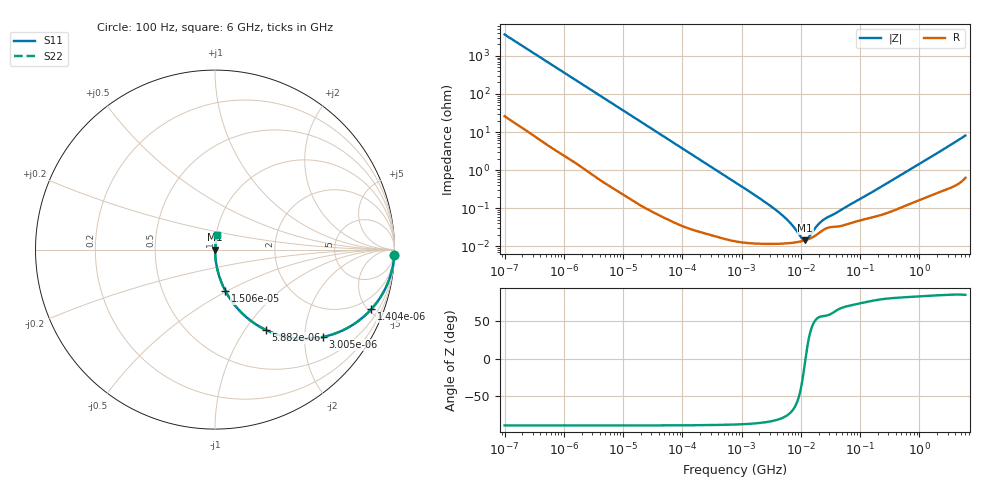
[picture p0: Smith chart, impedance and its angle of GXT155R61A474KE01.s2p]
!Murata Part Number: GXT155R61A474KE01
!These Parameters are Measured in Series Mode Connection
!Data Generated on Jan 08, 2026
!  o--ll--o
!Port1  Port2
!  o------o
!Operation Temp=25[degC], DC Bias Voltage=0[V]
!Freq. Start=100[Hz] Stop=6[GHz] 401[Steps]
# Hz S RI R 50
!Freq.(Hz) S11(Real) S11(Imag) S21(Real) S21(Imag) S12(Real) S12(Imag) S22(Real) S22(Imag)
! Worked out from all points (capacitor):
!   401 points, 100 Hz to 6 GHz, reference 50 ohm
!   read as one part in series: C = 438 nF near 109 Hz
!   lowest |Z| = 14.5 mohm at 11.89 MHz (marker M1)
!   series resonance near 12 MHz, so ESL is about 400 pH
!   S11 on the Smith chart (normalised r, x): 100 Hz: 2, -72; 1.404 kHz: 1.03, -5.22; 3.005 kHz: 1.02, -2.45; 5.882 kHz: 1.01, -1.25; 15.06 kHz: 1.00, -0.49; 6 GHz: 1.01, +0.16
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100  0.999 -0.0276  0.000958 0.0276  0.000958 0.0276  0.999 -0.0276
438  0.985 -0.1182  0.015 0.1182  0.015 0.1182  0.985 -0.1182
858  0.9466 -0.2216  0.0534 0.2216  0.0534 0.2216  0.9466 -0.2216
1404  0.8705 -0.3325  0.1295 0.3325  0.1295 0.3325  0.8705 -0.3325
2008  0.7682 -0.4187  0.2318 0.4187  0.2318 0.4187  0.7682 -0.4187
3005  0.599 -0.487  0.401 0.487  0.401 0.487  0.599 -0.487
5882  0.2832 -0.4475  0.7168 0.4475  0.7168 0.4475  0.2832 -0.4475
9204  0.1402 -0.3441  0.8598 0.3441  0.8598 0.3441  0.1402 -0.3441
15062  0.0582 -0.231  0.9418 0.231  0.9418 0.231  0.0582 -0.231
40335  0.00904 -0.0911  0.991 0.0911  0.991 0.0911  0.00904 -0.0911
129199  0.00112 -0.0288  0.9989 0.0288  0.9989 0.0288  0.00112 -0.0288
774597  0.000159 -0.00483  0.9998 0.00483  0.9998 0.00483  0.000159 -0.00483
4246196  0.000117 -0.000776  0.9999 0.000776  0.9999 0.000776  0.000117 -0.000776
6644369  0.000122 -0.000392  0.9999 0.000392  0.9999 0.000392  0.000122 -0.000392
1.039699e7  0.000137 -9e-05  0.9999 9e-05  0.9999 9e-05  0.000137 -9e-05
1.189169e7  0.000145 -5.7e-06  0.9999 5.7e-06  0.9999 5.7e-06  0.000145 -5.7e-06
1.300572e7  0.000152 5e-05  0.9998 -5e-05  0.9998 -5e-05  0.000152 5e-05
1.555665e7  0.000171 0.000162  0.9998 -0.000162  0.9998 -0.000162  0.000171 0.000162
2.035112e7  0.000224 0.000328  0.9998 -0.000328  0.9998 -0.000328  0.000224 0.000328
2.545746e7  0.000284 0.000443  0.9997 -0.000443  0.9997 -0.000443  0.000284 0.000443
3.124326e8  0.000808 0.00485  0.9992 -0.00485  0.9992 -0.00485  0.000808 0.00485
6e9  0.0125 0.079  0.9875 -0.079  0.9875 -0.079  0.0125 0.079
